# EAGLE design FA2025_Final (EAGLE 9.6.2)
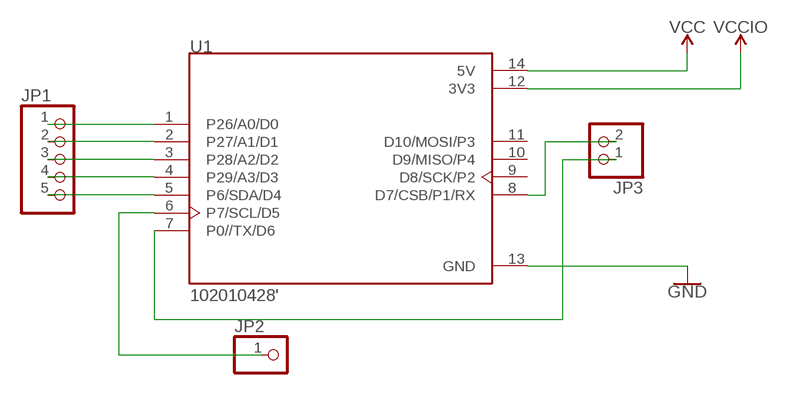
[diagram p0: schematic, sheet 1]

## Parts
JP1  PINHD-1X5  [1X05]
JP2  PINHD-1X1  [1X01]
JP3  PINHD-1X2  [1X02]
U1  102010428'  [MODULE_102010428]

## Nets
GND: U1.13(GND)
N$1: JP1.1 U1.1(P26/A0/D0)
N$2: JP1.2 U1.2(P27/A1/D1)
N$3: JP1.3 U1.3(P28/A2/D2)
N$4: JP1.4 U1.4(P29/A3/D3)
N$5: JP1.5 U1.5(P6/SDA/D4)
N$6: JP2.1 U1.6(P7/SCL/D5)
N$7: JP3.1 U1.7(P0//TX/D6)
N$8: JP3.2 U1.8(D7/CSB/P1/RX)
VCC: U1.14(5V)
VCCIO: U1.12(3V3)
Unconnected: U1.9(D8/SCK/P2) U1.10(D9/MISO/P4) U1.11(D10/MOSI/P3)

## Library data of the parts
JP1 = drazzy_pinhead:PINHD-1X5: PIN HEADER
JP2 = drazzy_pinhead:PINHD-1X1: PIN HEADER
JP3 = drazzy_pinhead:PINHD-1X2: PIN HEADER
U1 = 102010428:102010428: Check availability; AVAILABILITY: In Stock; CHECK_PRICES: https://www.snapeda.com/parts/102010428/Seeed+Studio/view-part/?ref=eda; DESCRIPTION: RP2040 XIAO RP2040 series ARM® Cortex®-M0+ MCU 32-Bit Embedded Evaluation Board; MF: Seeed Technology Co., Ltd; MP: 102010428; PACKAGE: None; PRICE: None; SNAPEDA_LINK: https://www.snapeda.com/parts/102010428/Seeed+Studio/view-part/?ref=snap

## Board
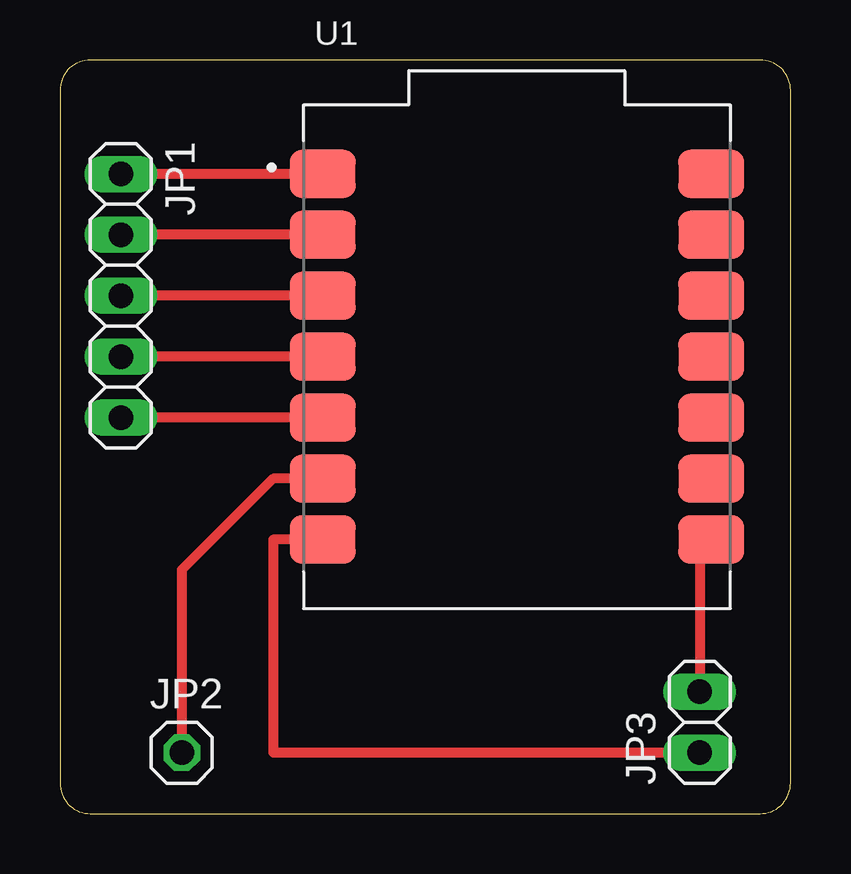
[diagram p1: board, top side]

Size 30.46 x 31.42 mm. Coordinates in mm from the lower left corner, seen from the top.
Outline: 0,30.15 0,1.27 arc90 1.27,0 29.19,0 arc90 30.46,1.27 30.46,30.15 arc90 29.19,31.42 1.27,31.42 arc90 0,30.15
Copper layers (1*16): Top 0.035mm / dielectric 1.5mm / Bottom 0.035mm
Design rules "default *": minimum track width 16mil, minimum drill 0.35mm, track to track 16mil, track to pad 16mil, pad to pad 16mil, via to via 16mil, smd to smd 24mil, copper to edge 40mil, drill to drill 6mil, minimum pad ring 10mil, minimum via ring 8mil, stop-mask expansion 4mil, vias tented up to drill 0mil, thermal gap 10mil

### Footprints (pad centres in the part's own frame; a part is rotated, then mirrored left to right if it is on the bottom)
1X05 = drill 1.016 long: 1 -5.08,0; 2 -2.54,0; 3 0,0; 4 2.54,0; 5 5.08,0
1X01 = drill 1.016 octagon: 1 0,0
1X02 = drill 1.016 long: 1 -1.27,0; 2 1.27,0
MODULE_102010428 = smd 2.75 x 2: 1 -8.1,7.62; 2 -8.1,5.08; 3 -8.1,2.54; 4 -8.1,0; 5 -8.1,-2.54; 6 -8.1,-5.08; 7 -8.1,-7.62; 8 8.1,-7.62; 9 8.1,-5.08; 10 8.1,-2.54; 11 8.1,0; 12 8.1,2.54; 13 8.1,5.08; 14 8.1,7.62

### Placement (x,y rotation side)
JP1  2.54,21.59 270 top
JP2  5.08,2.54 0 top
JP3  26.67,3.81 90 top
U1  19.05,19.05 0 top

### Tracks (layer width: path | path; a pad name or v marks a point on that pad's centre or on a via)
N$1
  Top 0.406: U1.1 JP1.1
N$2
  Top 0.406: U1.2 JP1.2
N$3
  Top 0.406: U1.3 JP1.3
N$4
  Top 0.406: U1.4 JP1.4
N$5
  Top 0.406: U1.5 JP1.5
N$6
  Top 0.406: U1.6 8.89,13.97 5.08,10.16 JP2.1
N$7
  Top 0.406: U1.7 8.89,11.43 8.89,2.54 JP3.1
N$8
  Top 0.406: U1.8 26.67,10.95 JP3.2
